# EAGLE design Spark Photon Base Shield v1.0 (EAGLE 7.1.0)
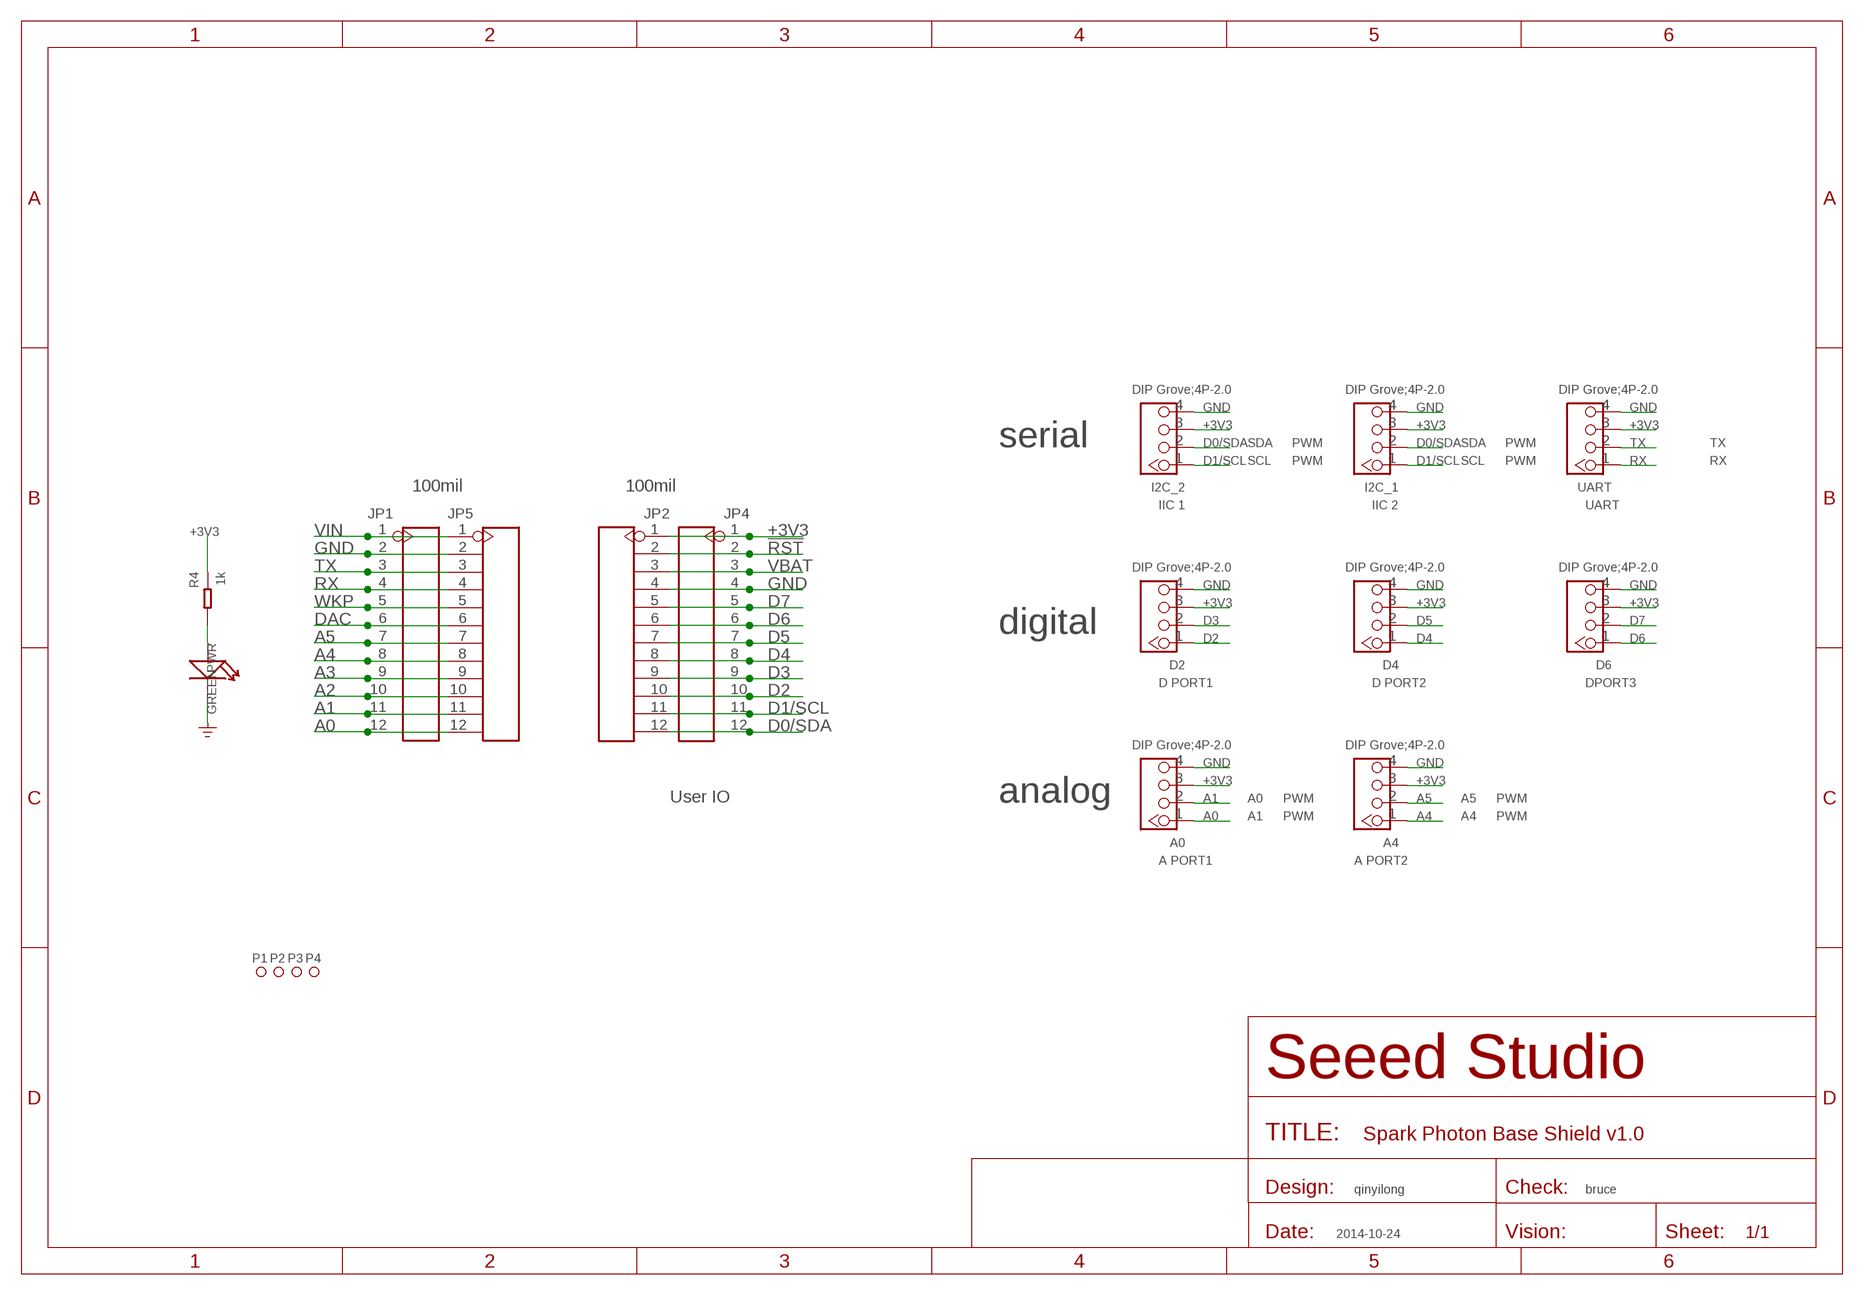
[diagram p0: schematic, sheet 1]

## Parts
A0  DIP Grove;4P-2.0  TWIG-4P-2.0-2.0  [4P-2.0]
A4  DIP Grove;4P-2.0  TWIG-4P-2.0-2.0  [4P-2.0]
D2  DIP Grove;4P-2.0  TWIG-4P-2.0-2.0  [4P-2.0]
D4  DIP Grove;4P-2.0  TWIG-4P-2.0-2.0  [4P-2.0]
D6  DIP Grove;4P-2.0  TWIG-4P-2.0-2.0  [4P-2.0]
I2C_1  DIP Grove;4P-2.0  TWIG-4P-2.0-2.0  [4P-2.0]
I2C_2  DIP Grove;4P-2.0  TWIG-4P-2.0-2.0  [4P-2.0]
JP1  HEADER-12P-2.54  [12P-2.54-65/35MIL]
JP2  HEADER-12P-2.54  [12P-2.54-65/35MIL]
JP4  HEADER-12P-2.54  [12P-2.54-65/35MIL]
JP5  HEADER-12P-2.54  [12P-2.54-65/35MIL]
P1  MARK-1.0'ANNULAR'  [ROUND-MARK-1.0]
P2  MARK-1.0'ANNULAR'  [ROUND-MARK-1.0]
P3  MARK-1.0'ANNULAR'  [ROUND-MARK-1.0]
P4  MARK-1.0'ANNULAR'  [ROUND-MARK-1.0]
PWR  GREEN  LED'0603'  [LED-0603]
R4  1k  RES-0603  [R0603]
UART  DIP Grove;4P-2.0  TWIG-4P-2.0-2.0  [4P-2.0]

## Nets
!RST: JP2.2 JP4.2
+3V3: A0.3 A4.3 D2.3 D4.3 D6.3 I2C_1.3 I2C_2.3 JP2.1 JP4.1 R4.1 UART.3
A0: A0.1 JP1.12 JP5.12
A1: A0.2 JP1.11 JP5.11
A2: JP1.10 JP5.10
A3: JP1.9 JP5.9
A4: A4.1 JP1.8 JP5.8
A5: A4.2 JP1.7 JP5.7
D0/SDA: I2C_1.2 I2C_2.2 JP2.12 JP4.12
D1/SCL: I2C_1.1 I2C_2.1 JP2.11 JP4.11
D2: D2.1 JP2.10 JP4.10
D3: D2.2 JP2.9 JP4.9
D4: D4.1 JP2.8 JP4.8
D5: D4.2 JP2.7 JP4.7
D6: D6.1 JP2.6 JP4.6
D7: D6.2 JP2.5 JP4.5
DAC: JP1.6 JP5.6
GND: A0.4 A4.4 D2.4 D4.4 D6.4 I2C_1.4 I2C_2.4 JP1.2 JP2.4 JP4.4 JP5.2 PWR.- UART.4 ; supply symbol labelled GND_POWER
N$1: PWR.+ R4.2
RX: JP1.4 JP5.4 UART.1
TX: JP1.3 JP5.3 UART.2
VBAT: JP2.3 JP4.3
VIN: JP1.1 JP5.1
WKP: JP1.5 JP5.5

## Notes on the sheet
- serial | SDA | PWM | SDA | PWM | TX
- SCL | PWM | SCL | PWM | RX
- 100mil | 100mil
- IIC 1 | IIC 2 | UART
- digital
- D PORT1 | D PORT2 | DPORT3
- User IO | analog | A0 | PWM | A5 | PWM
- A1 | PWM | A4 | PWM
- A PORT1 | A PORT2
- qinyilong | bruce
- 2014-10-24

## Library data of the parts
A0 A4 D2 D4 D6 I2C_1 I2C_2 UART = Connector:TWIG-4P-2.0
JP1 JP2 JP4 JP5 = Connector-new:HEADER-12P
P1-P4 = Discrete-new:MARK-1.0; PARTNO: DNP
PWR = Discrete:LED*
R4 = Discrete-new:RES

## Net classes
0 default: width 0.203 mm, drill 0.305 mm, clearance 0.127 mm

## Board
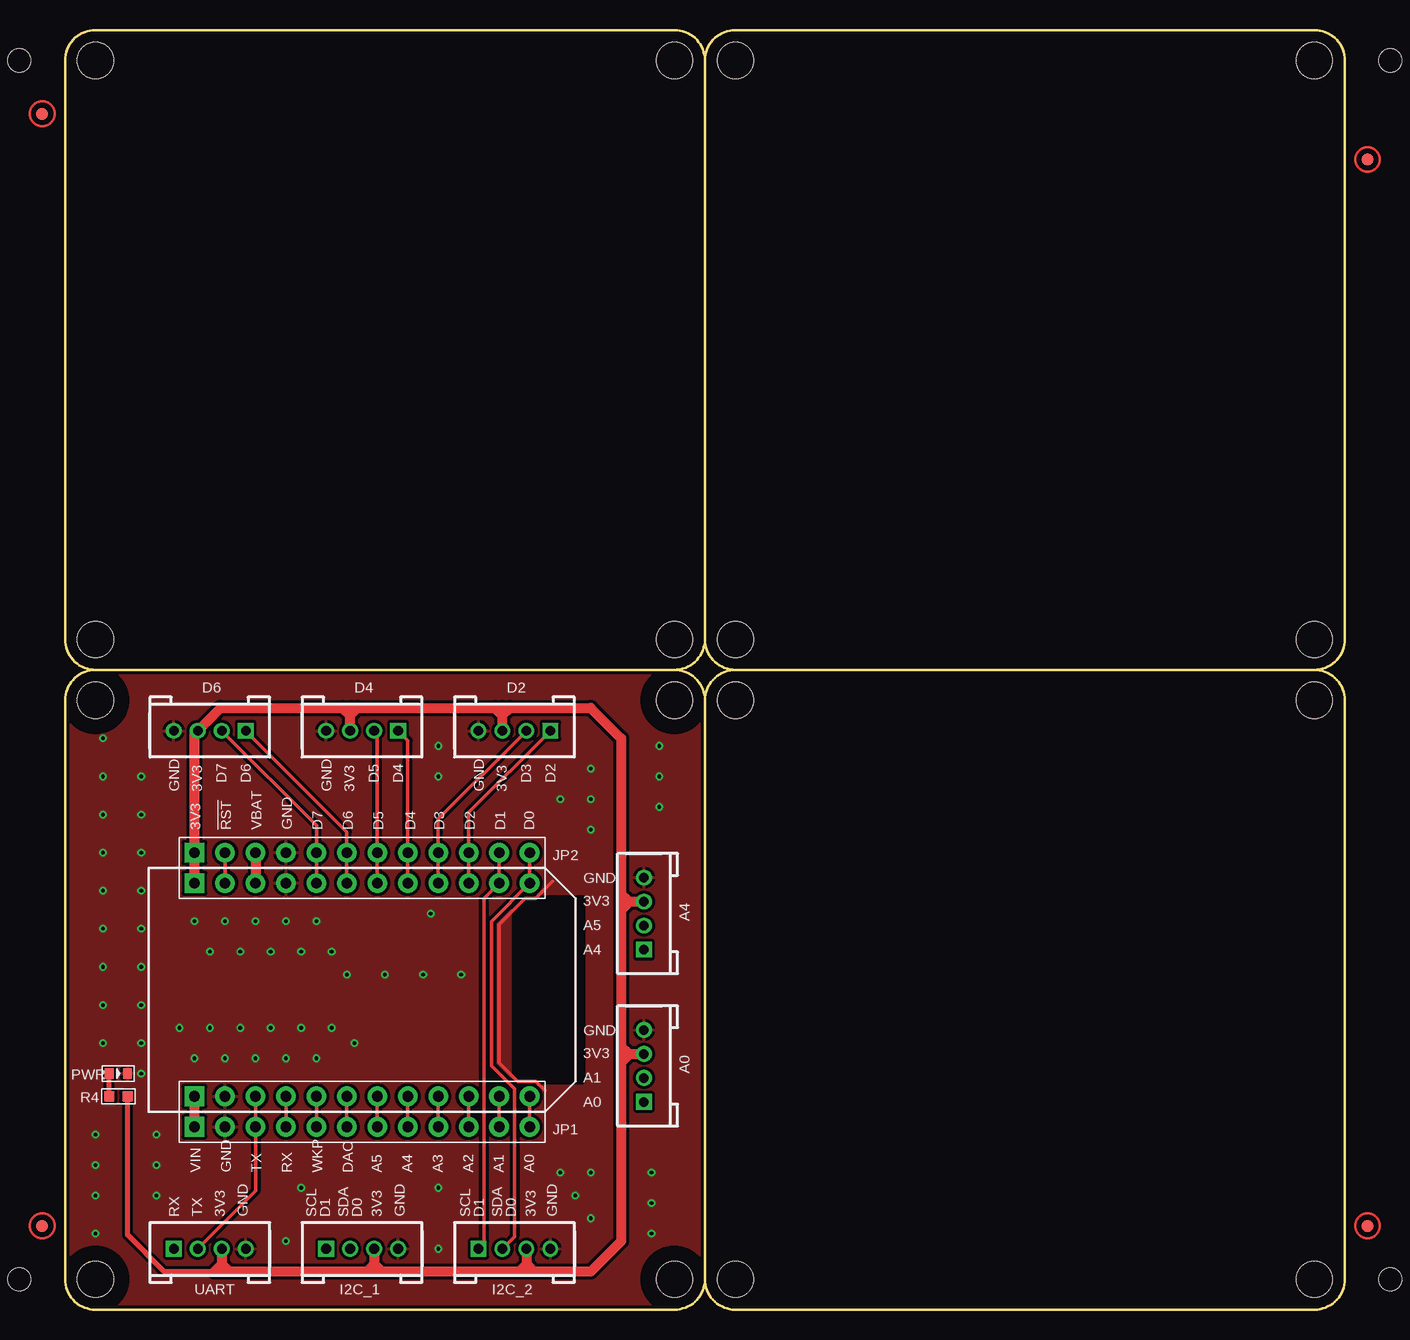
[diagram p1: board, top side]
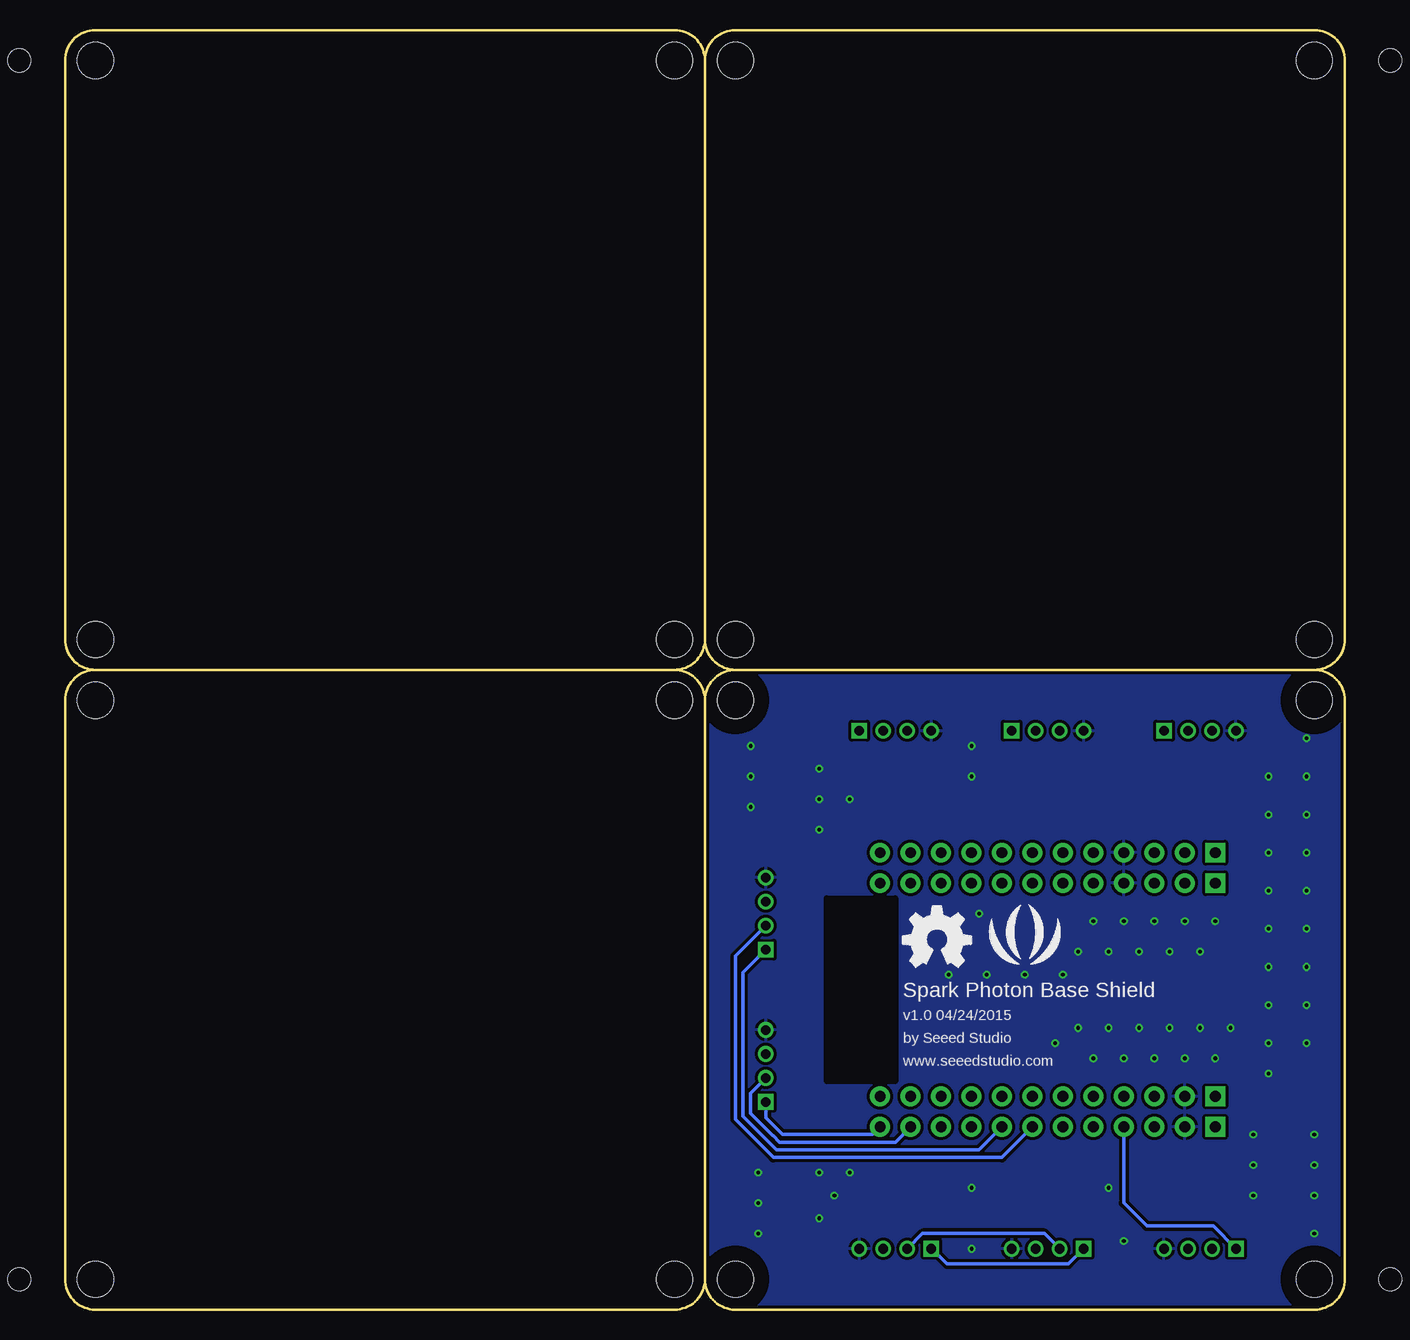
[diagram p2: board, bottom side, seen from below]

Size 106.68 x 106.68 mm. Coordinates in mm from the lower left corner, seen from the top.
Outline: 2.54,53.34 arc90 0,50.8 0,2.54 arc90 2.54,0 50.8,0 arc90 53.34,2.54
Outline: 50.8,53.34 arc-90 53.34,50.8
Outline: 53.34,2.54 arc90 55.88,0 104.14,0 arc90 106.68,2.54 106.68,50.8 arc90 104.14,53.34
Outline: 53.34,2.54 53.34,50.8
Outline: 53.34,50.8 arc-90 55.88,53.34
Outline: 50.8,53.34 2.54,53.34
Outline: 2.54,53.34 arc-90 0,55.88 0,104.14 arc-90 2.54,106.68 50.8,106.68 arc-90 53.34,104.14
Outline: 53.34,55.88 arc-90 50.8,53.34
Outline: 104.14,53.34 55.88,53.34
Outline: 55.88,53.34 arc-90 53.34,55.88
Outline: 53.34,55.88 53.34,104.14
Outline: 53.34,104.14 arc-90 55.88,106.68 104.14,106.68 arc-90 106.68,104.14 106.68,55.88 arc-90 104.14,53.34
Copper layers (1*16): Top 0.035mm / dielectric 1.5mm / Bottom 0.035mm
Design rules "SeeedStudio_rule_no_angle_090911 *": minimum track width 6mil, minimum drill 12mil, track to track 6mil, track to pad 6mil, pad to pad 6mil, via to via 6mil, smd to smd 0mil, copper to edge 10mil, drill to drill 10mil, minimum pad ring 10mil, minimum via ring 6mil, stop-mask expansion 2mil, vias tented up to drill 100mil, thermal gap 10mil
Holes 3 mm at 2.54,50.8 50.8,50.8 50.8,2.54 2.54,2.54 55.88,50.8 104.14,50.8 104.14,2.54 55.88,2.54 2.54,104.14 50.8,104.14 50.8,55.88 2.54,55.88 55.88,104.14 104.14,104.14 104.14,55.88 55.88,55.88
Holes 1.91 mm at -3.81,2.54 -3.81,104.14 110.49,104.14 110.49,2.54
tRestrict: area 0,0 to 5.1,5.1; area 48.2,0 to 53.4,5.1; area 48.2,48.2 to 53.4,53.4; area 0,48.2 to 5.1,53.4; area 37.5,19.1 to 43.2,34.3
bRestrict: area 0,0 to 5.1,5.1; area 48.2,0 to 53.4,5.1; area 48.2,48.2 to 53.4,53.4; area 0,48.2 to 5.1,53.4; area 37.5,19.1 to 43.2,34.3

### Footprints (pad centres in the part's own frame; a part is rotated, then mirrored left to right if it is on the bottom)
4P-2.0 = drill 0.8 pad 1.27 square: 1 -3,0 | drill 0.8 pad 1.27: 2 -1,0; 3 1,0; 4 3,0
12P-2.54-65/35MIL = drill 0.889 pad 1.651 square: 1 0,13.97 | drill 0.889 pad 1.651: 2 0,11.43; 3 0,8.89; 4 0,6.35; 5 0,3.81; 6 0,1.27; 7 0,-1.27; 8 0,-3.81; 9 0,-6.35; 10 0,-8.89; 11 0,-11.43; 12 0,-13.97
ROUND-MARK-1.0 = smd 1.016 x 1.016: P$1 0,0
LED-0603 = smd 0.762 x 0.889: + -0.762,0; - 0.762,0
R0603 = smd 0.889 x 0.889: 1 -0.762,0; 2 0.762,0

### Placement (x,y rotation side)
A0  48.26,20.32 90 top
A4  48.26,33.02 90 top
D2  37.47,48.26 180 top
D4  24.77,48.26 180 top
D6  12.06,48.26 180 top
I2C_1  24.77,5.08 0 top
I2C_2  37.47,5.08 0 top
JP1  24.77,15.24 90 top
JP2  24.77,38.1 90 top
JP4  24.77,35.56 90 top
JP5  24.77,17.78 90 top
P1  -1.91,6.99 0 top
P2  -1.91,99.69 0 top
P3  108.58,6.99 0 top
P4  108.58,95.89 0 top
PWR  4.45,19.68 0 top
R4  4.45,17.78 180 top
U$1  [OSHW_FILLX200_NOTEXT]  36.83,28.57 0 bottom
U$2  [SEEED-SILK-280*268MIL]  26.67,30.48 0 bottom
UART  12.06,5.08 0 top

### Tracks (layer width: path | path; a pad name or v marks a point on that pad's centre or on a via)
!RST
  Top 0.305: JP4.2 JP2.2
+3V3
  Top 0.406: 12.45,3.17 8.26,3.17 5.21,6.22 R4.1
  Top 0.813: JP4.1 JP2.1 10.79,47.99 D6.3 12.97,50.16 | 12.95,50.16 12.97,50.16 | 12.97,50.16 23.11,50.16 | 23.11,50.16 23.88,50.16 | 23.88,50.16 24.38,50.16 | 24.38,50.16 35.81,50.16 | 35.81,50.16 36.45,50.16 | 36.45,50.16 37.08,50.16 | 37.08,50.16 43.81,50.16 46.35,47.62 46.35,34.67 | 46.35,34.67 46.35,34.16 | 46.35,34.16 46.35,34.04 | 46.35,34.04 46.35,33.27 | 46.35,33.27 46.35,21.97 | 46.35,21.97 46.35,21.34 | 46.35,21.34 46.35,20.57 | 46.35,20.57 46.35,5.71 43.81,3.17 39.12,3.17 | 39.12,3.17 38.48,3.17 | 38.48,3.17 37.85,3.17 | 37.85,3.17 26.42,3.17 | 26.42,3.17 25.78,3.17 | 25.78,3.17 25.15,3.17 | 25.15,3.17 13.72,3.17 | 13.72,3.17 13.08,3.17 | 13.08,3.17 12.45,3.17 13.06,3.79 | UART.3 13.06,3.83 | 13.06,3.79 13.06,3.19 13.08,3.17 | I2C_2.3 38.47,3.79 | 38.47,3.79 38.47,3.19 38.48,3.17 | I2C_1.3 25.77,3.83 | 25.77,3.79 25.77,3.19 25.78,3.17 | 13.06,3.83 13.72,3.17 | 13.06,3.83 13.06,3.79 | 25.77,3.83 26.42,3.17 | 25.77,3.83 25.77,3.79 | 25.77,3.79 25.15,3.17 | 38.47,3.79 37.85,3.17 | 38.47,3.79 38.5,3.79 39.12,3.17 | 46.37,34.02 46.35,34.04 | D2.3 36.47,50.15 36.45,50.16 | 35.81,50.16 36.45,49.53 37.08,50.16 | D4.3 23.77,50.05 23.88,50.16 | 23.11,50.16 23.75,49.53 24.38,50.16 | 47.01,34.02 46.5,34.02 46.35,34.16 | 47.01,21.32 46.37,21.32 46.35,21.34 | 47.1,21.32 47.01,21.32 | 47.01,21.32 46.35,21.97 | 47.1,21.32 46.35,20.57 | 47.1,34.02 47.01,34.02 | 47.01,34.02 46.35,34.67 | 47.1,34.02 46.35,33.27 | 47.1,21.32 A0.3 | 47.1,34.02 A4.3
A0
  Top 0.305: JP1.12 JP5.12
  Bottom 0.305: JP1.12 39.37,14.61 46.86,14.61 48.26,16 A0.1
A1
  Top 0.305: JP1.11 JP5.11
  Bottom 0.305: JP1.11 37.47,13.97 47.12,13.97 47.62,14.48 47.69,14.54 49.53,16.38 49.53,18.05 A0.2
A2
  Top 0.305: JP1.10 JP5.10
A3
  Top 0.305: JP1.9 JP5.9
A4
  Top 0.305: JP1.8 JP5.8
  Bottom 0.305: JP1.8 30.48,13.34 47.37,13.34 49.78,15.75 49.91,15.88 50.16,16.13 50.16,28.11 A4.1
A5
  Top 0.305: JP1.7 JP5.7
  Bottom 0.305: JP1.7 28.57,12.7 47.62,12.7 50.8,15.88 50.8,29.48 50.16,30.11 50.11,30.17 A4.2
D0/SDA
  Top 0.305: JP2.12 JP4.12 35.56,32.38 35.56,20.32 37.47,18.41 37.47,6.08 I2C_2.2
  Bottom 0.305: I2C_1.2 25.04,6.35 35.2,6.35 I2C_2.2 36.45,5.08
D1/SCL
  Top 0.305: JP2.11 JP4.11 34.92,34.29 34.92,5.54 I2C_2.1
  Bottom 0.305: I2C_2.1 34.42,5.08 33.15,3.81 23.04,3.81 I2C_1.1
D2
  Top 0.305: JP4.10 JP2.10 33.66,41.45 D2.1
D3
  Top 0.305: JP4.9 JP2.9 31.11,40.91 D2.2
D4
  Top 0.305: JP4.8 JP2.8 28.57,47.45 D4.1
D5
  Top 0.305: JP4.7 JP2.7 26.04,47.99 D4.2
D6
  Top 0.305: JP4.6 JP2.6 23.5,39.83 D6.1
D7
  Top 0.305: JP4.5 JP2.5 20.95,40.37 D6.2
DAC
  Top 0.305: JP1.6 JP5.6
GND  (via drill 0.3 pad 0.64)
  Top 0.305: 40.01,18.29 39.24,19.05 37.72,19.05 36.2,20.57 36.2,32.13 38.35,34.29 39.24,34.29 40.64,35.69
  other vias: 15.88,20.95 17.14,23.5 23.5,27.94 33.02,27.94 13.34,32.38 15.88,32.38 18.41,32.38 6.35,19.68 6.35,22.23 6.35,38.1 18.41,20.95 20.95,20.95 14.61,23.5 12.06,23.5 22.23,23.5 20.95,32.38 24.13,22.23 19.68,23.5 10.79,20.95 12.06,29.84 13.34,20.95 10.79,32.38 3.17,22.23 3.17,25.4 3.17,28.57 3.17,31.75 3.17,34.92 3.17,38.1 3.17,41.27 3.17,44.45 3.17,47.62 6.35,44.45 6.35,41.27 6.35,25.4 6.35,28.57 6.35,31.75 6.35,34.92 49.53,46.99 49.53,44.45 49.53,41.91 48.9,11.43 48.9,8.89 48.9,6.35 43.81,11.43 41.27,11.43 42.55,9.53 43.81,7.62 43.81,45.09 43.81,42.55 43.81,40.01 41.27,42.55 31.11,46.99 31.11,44.45 31.11,10.16 19.68,10.16 18.41,5.71 31.11,5.08 2.54,14.61 2.54,12.06 2.54,9.53 2.54,6.35 7.62,14.61 7.62,12.06 7.62,9.53 14.61,29.84 17.14,29.84 19.68,29.84 22.23,29.84 9.53,23.5 30.48,33.02 29.84,27.94 26.67,27.94
  pour Bottom (isolate 0.254, rank 6): 0,0 53.34,0 53.34,53.34 0,53.34
  pour Top (isolate 0.254, rank 6): 0,0 53.34,0 53.34,53.34 0,53.34
N$1
  Top 0.406: R4.2 PWR.+
RX
  Top 0.305: JP1.4 JP5.4
  Bottom 0.305: JP1.4 18.41,8.89 16.51,6.99 10.97,6.99 UART.1
TX
  Top 0.305: JP5.3 JP1.3 15.88,9.89 UART.2
VBAT
  Top 0.813: JP2.3 JP4.3 16.13,35.31
VIN
  Top 0.813: JP1.1 JP5.1
WKP
  Top 0.305: JP1.5 JP5.5

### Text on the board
tPlace: D7 | D6 | D5 | D4 | D3 | D2 | GND | 3V3 | GND | 3V3 | GND | 3V3 | 3V3 | !RST | VBAT | GND | D7 | D6 | D5 | D4 | D3 | D2 | D1 | D0 | GND | 3V3 | A5 | A4 | GND | 3V3 | A1 | A0 | VIN | GND | TX | RX | WKP | DAC | A5 | A4 | A3 | A2 | A1 | A0 | RX | TX | 3V3 | GND | SCL | D1 | SDA | D0 | 3V3 | GND | SCL | D1 | SDA | D0 | 3V3 | GND
bPlace: Spark Photon Base Shield | v1.0 04/24/2015 | by Seeed Studio | www.seeedstudio.com
bPlate: A0 | A2 | A4 | SPI | UART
